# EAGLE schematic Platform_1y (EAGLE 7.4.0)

## Sheet 1 of 5: Propeller
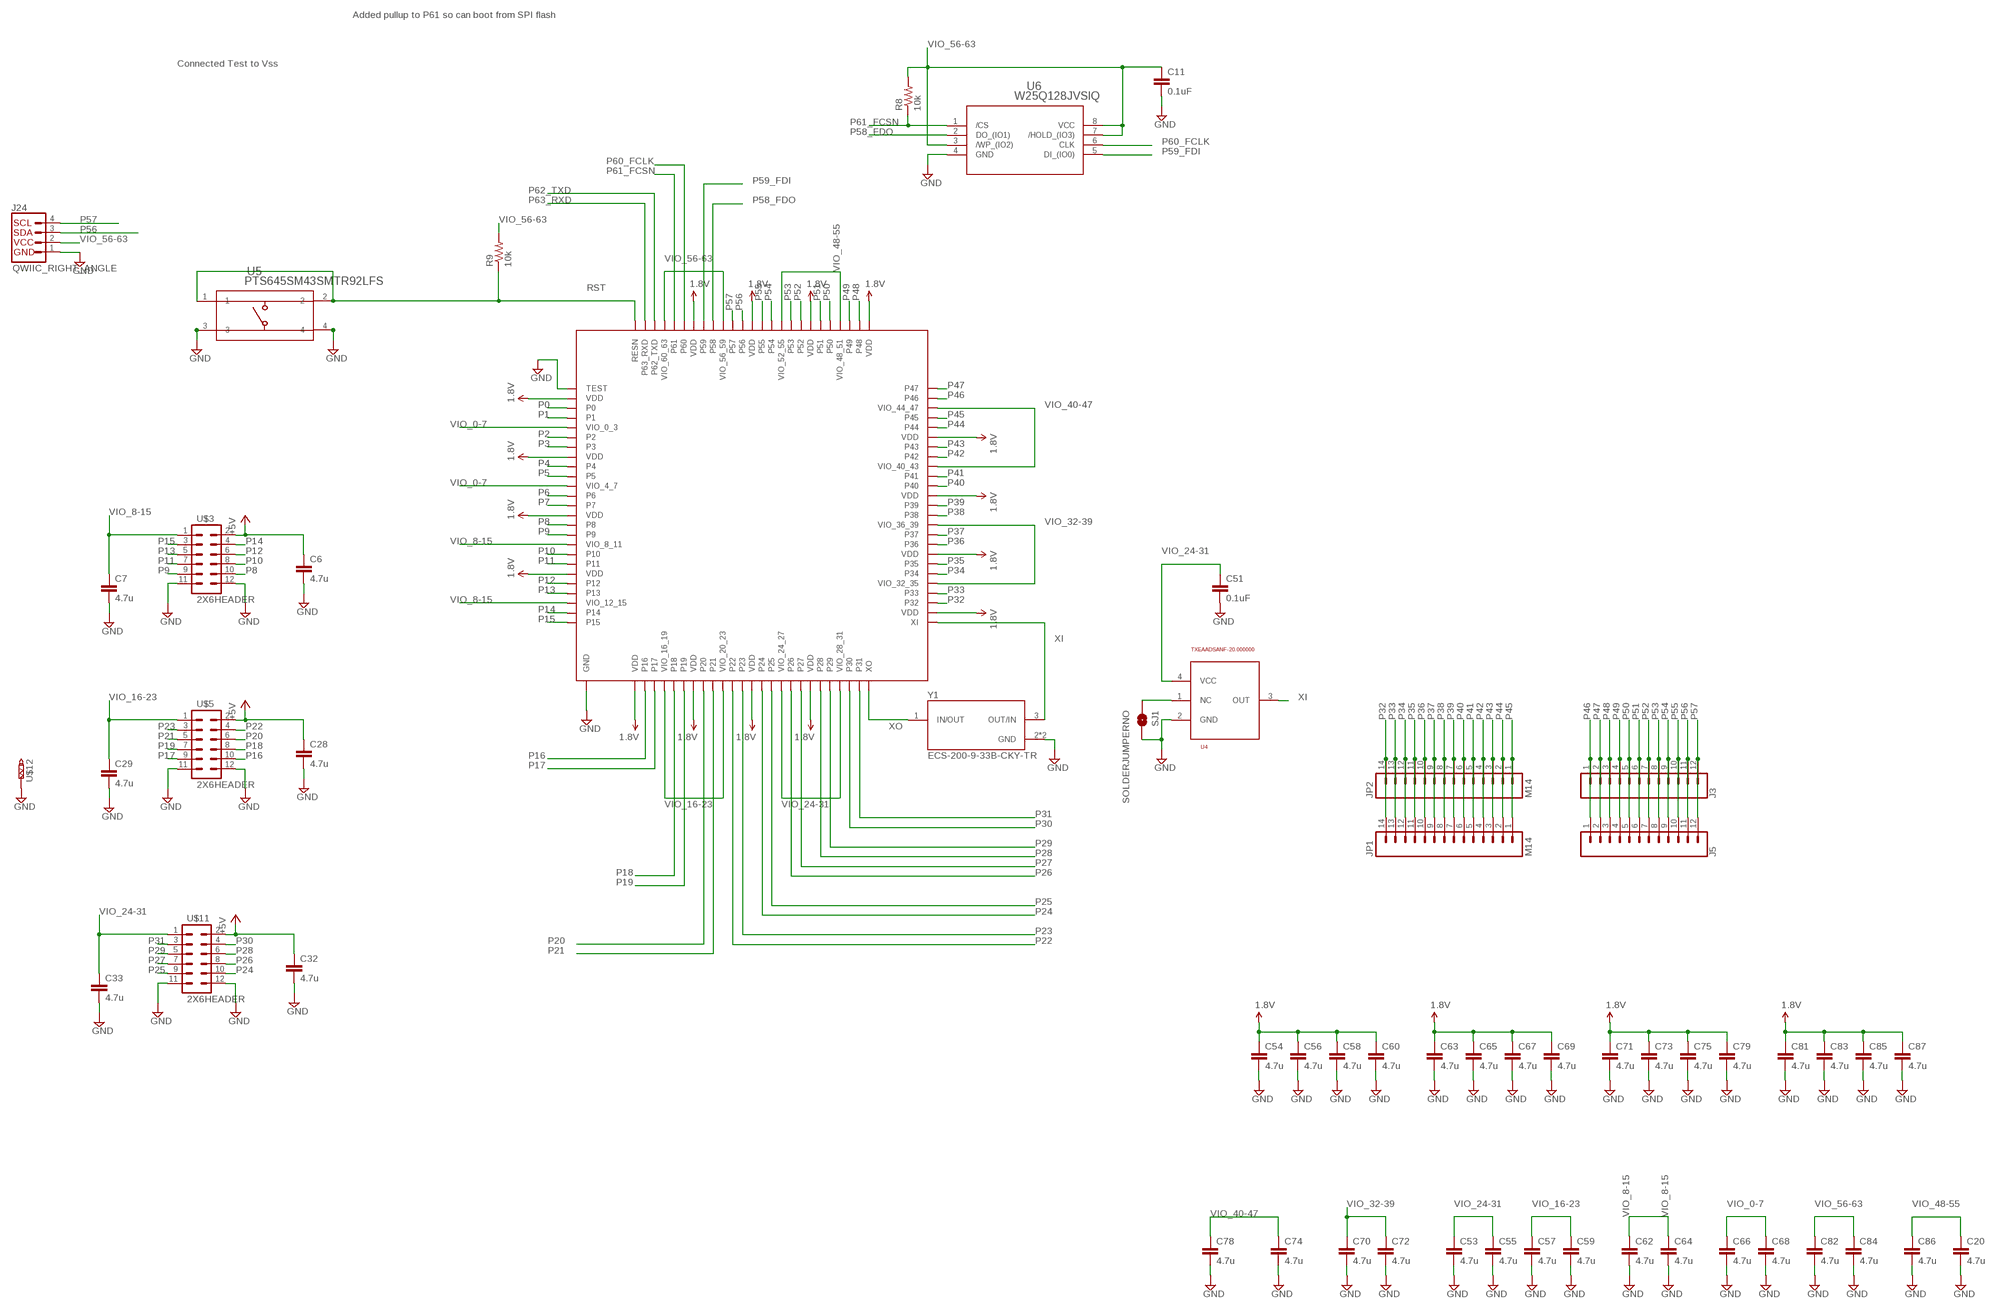
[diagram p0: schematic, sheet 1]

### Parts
C6  4.7u  2.2UF-CERCAP-07888  [0402-CAP]
C7  4.7u  2.2UF-CERCAP-07888  [0402-CAP]
C11  0.1uF  1.0UF-25V-+80/-20(0805)  [0805]
C20  4.7u  2.2UF-CERCAP-07888  [0402-CAP]
C28  4.7u  2.2UF-CERCAP-07888  [0402-CAP]
C29  4.7u  2.2UF-CERCAP-07888  [0402-CAP]
C32  4.7u  2.2UF-CERCAP-07888  [0402-CAP]
C33  4.7u  2.2UF-CERCAP-07888  [0402-CAP]
C51  0.1uF  22UF-6.3V-20%(0805)  [0805]
C53  4.7u  2.2UF-CERCAP-07888  [0402-CAP]
C54  4.7u  2.2UF-CERCAP-07888  [0402-CAP]
C55  4.7u  2.2UF-CERCAP-07888  [0402-CAP]
C56  4.7u  2.2UF-CERCAP-07888  [0402-CAP]
C57  4.7u  2.2UF-CERCAP-07888  [0402-CAP]
C58  4.7u  2.2UF-CERCAP-07888  [0402-CAP]
C59  4.7u  2.2UF-CERCAP-07888  [0402-CAP]
C60  4.7u  2.2UF-CERCAP-07888  [0402-CAP]
C62  4.7u  2.2UF-CERCAP-07888  [0402-CAP]
C63  4.7u  2.2UF-CERCAP-07888  [0402-CAP]
C64  4.7u  2.2UF-CERCAP-07888  [0402-CAP]
C65  4.7u  2.2UF-CERCAP-07888  [0402-CAP]
C66  4.7u  2.2UF-CERCAP-07888  [0402-CAP]
C67  4.7u  2.2UF-CERCAP-07888  [0402-CAP]
C68  4.7u  2.2UF-CERCAP-07888  [0402-CAP]
C69  4.7u  2.2UF-CERCAP-07888  [0402-CAP]
C70  4.7u  2.2UF-CERCAP-07888  [0402-CAP]
C71  4.7u  2.2UF-CERCAP-07888  [0402-CAP]
C72  4.7u  2.2UF-CERCAP-07888  [0402-CAP]
C73  4.7u  2.2UF-CERCAP-07888  [0402-CAP]
C74  4.7u  2.2UF-CERCAP-07888  [0402-CAP]
C75  4.7u  2.2UF-CERCAP-07888  [0402-CAP]
C78  4.7u  2.2UF-CERCAP-07888  [0402-CAP]
C79  4.7u  2.2UF-CERCAP-07888  [0402-CAP]
C81  4.7u  2.2UF-CERCAP-07888  [0402-CAP]
C82  4.7u  2.2UF-CERCAP-07888  [0402-CAP]
C83  4.7u  2.2UF-CERCAP-07888  [0402-CAP]
C84  4.7u  2.2UF-CERCAP-07888  [0402-CAP]
C85  4.7u  2.2UF-CERCAP-07888  [0402-CAP]
C86  4.7u  2.2UF-CERCAP-07888  [0402-CAP]
C87  4.7u  2.2UF-CERCAP-07888  [0402-CAP]
J3  CONN_12  [1X12]
J5  CONN_12  [1X12]
J24  QWIIC_RIGHT_ANGLE  QWIIC_CONNECTORJS-1MM  [JST04_1MM_RA]
JP1  M14  [1X14]
JP2  M14  [1X14]
R8  10k  0.75OHM1/4W1%(0805)  [0805]
R9  10k  0.75OHM1/4W1%(0805)  [0805]
SJ1  SOLDERJUMPERNO  [SJ_2S-NO]
U2  Propeller 2 - ES  P2X8C4M64P-ES_  [PROPELLER_2]
U4  TXEAADSANF-20.000000  [3.2X2.5_4SMD]
U5  PTS645SM43SMTR92LFS  [SWITCH_43SMTR92LFS]
U6  W25Q128JVSIQ  [SOIC_128JVSIQ_WIN]
U$3  2X6HEADER  [6X2HEADER]
U$5  2X6HEADER  [6X2HEADER]
U$11  2X6HEADER  [6X2HEADER]
U$12  TURRET-1520PTH  [1X01_TURRET]
Y1  ECS-200-9-33B-CKY-TR  [XTAL_ECS-200-9-33B-CKY-TR]

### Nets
1.8V: C54.1 C56.1 C58.1 C60.1 C63.1 C65.1 C67.1 C69.1 C71.1 C73.1 C75.1 C79.1 C81.1 C83.1 C85.1 C87.1 U2.2(VDD) U2.8(VDD) U2.14(VDD) U2.20(VDD) U2.26(VDD) U2.32(VDD) U2.38(VDD) U2.44(VDD) U2.52(VDD) U2.58(VDD) U2.64(VDD) U2.70(VDD) U2.76(VDD) U2.82(VDD) U2.88(VDD) U2.94(VDD) ; also sheet 2,4
+5V: C6.1 C28.1 C32.1 U$3.2 U$5.2 U$11.2 ; also sheet 2,4
GND [gnd]: C6.2 C7.2 C11.2 C20.2 C28.2 C29.2 C32.2 C33.2 C51.2 C53.2 C54.2 C55.2 C56.2 C57.2 C58.2 C59.2 C60.2 C62.2 C63.2 C64.2 C65.2 C66.2 C67.2 C68.2 C69.2 C70.2 C71.2 C72.2 C73.2 C74.2 C75.2 C78.2 C79.2 C81.2 C82.2 C83.2 C84.2 C85.2 C86.2 C87.2 J24.1 SJ1.2 U2.1(TEST) U2.EP(GND) U4.2(GND) U5.3 U5.4 U6.4(GND) U$3.11 U$3.12 U$5.11 U$5.12 U$11.11 U$11.12 U$12.1 Y1.2(GND) Y1.4(GND) ; also sheet 2,3,4
N$1 [power]: SJ1.1 U4.1(NC)
P0: U2.3(P0) ; also sheet 3
P1: U2.4(P1) ; also sheet 3
P2: U2.6(P2) ; also sheet 3
P3: U2.7(P3) ; also sheet 3
P4: U2.9(P4) ; also sheet 3
P5: U2.10(P5) ; also sheet 3
P6: U2.12(P6) ; also sheet 3
P7: U2.13(P7) ; also sheet 3
P8: U2.15(P8) U$3.10
P9: U2.16(P9) U$3.9
P10: U2.18(P10) U$3.8
P11: U2.19(P11) U$3.7
P12: U2.21(P12) U$3.6
P13: U2.22(P13) U$3.5
P14: U2.24(P14) U$3.4
P15: U2.25(P15) U$3.3
P16: U2.27(P16) U$5.10
P17: U2.28(P17) U$5.9
P18: U2.30(P18) U$5.8
P19: U2.31(P19) U$5.7
P20: U2.33(P20) U$5.6
P21: U2.34(P21) U$5.5
P22: U2.36(P22) U$5.4
P23: U2.37(P23) U$5.3
P24: U2.39(P24) U$11.10
P25: U2.40(P25) U$11.9
P26: U2.42(P26) U$11.8
P27: U2.43(P27) U$11.7
P28: U2.45(P28) U$11.6
P29: U2.46(P29) U$11.5
P30: U2.48(P30) U$11.4
P31: U2.49(P31) U$11.3
P32: JP1.14 JP2.14 U2.53(P32) ; also sheet 3
P33: JP1.13 JP2.13 U2.54(P33) ; also sheet 3
P34: JP1.12 JP2.12 U2.56(P34) ; also sheet 3
P35: JP1.11 JP2.11 U2.57(P35) ; also sheet 3
P36: JP1.10 JP2.10 U2.59(P36) ; also sheet 3
P37: JP1.9 JP2.9 U2.60(P37) ; also sheet 3
P38: JP1.8 JP2.8 U2.62(P38) ; also sheet 3
P39: JP1.7 JP2.7 U2.63(P39) ; also sheet 3
P40: JP1.6 JP2.6 U2.65(P40) ; also sheet 3
P41: JP1.5 JP2.5 U2.66(P41) ; also sheet 3
P42: JP1.4 JP2.4 U2.68(P42) ; also sheet 3
P43: JP1.3 JP2.3 U2.69(P43) ; also sheet 3
P44: JP1.2 JP2.2 U2.71(P44) ; also sheet 3
P45: JP1.1 JP2.1 U2.72(P45) ; also sheet 3
P46: J3.1 J5.1 U2.74(P46) ; also sheet 3
P47: J3.2 J5.2 U2.75(P47) ; also sheet 3
P48: J3.3 J5.3 U2.77(P48) ; also sheet 3
P49: J3.4 J5.4 U2.78(P49) ; also sheet 3
P50: J3.5 J5.5 U2.80(P50) ; also sheet 3
P51: J3.6 J5.6 U2.81(P51) ; also sheet 3
P52: J3.7 J5.7 U2.83(P52)
P53: J3.8 J5.8 U2.84(P53)
P54: J3.9 J5.9 U2.86(P54)
P55: J3.10 J5.10 U2.87(P55)
P56: J3.11 J5.11 J24.3 U2.89(P56)
P57: J3.12 J5.12 J24.4 U2.90(P57)
P58_FDO: U2.92(P58) U6.2(DO_(IO1))
P59_FDI: U2.93(P59) U6.5(DI_(IO0))
P60_FCLK: U2.95(P60) U6.6(CLK)
P61_FCSN: R8.1 U2.96(P61) U6.1(/CS)
P62_TXD: U2.98(P62_TXD) ; also sheet 2
P63_RXD: U2.99(P63_RXD) ; also sheet 2
RST: R9.1 U2.100(RESN) U5.1 U5.2 ; also sheet 2
VIO_0-7: C66.1 C68.1 U2.5(VIO_0_3) U2.11(VIO_4_7) ; also sheet 3,4
VIO_8-15: C7.1 C62.1 C64.1 U2.17(VIO_8_11) U2.23(VIO_12_15) U$3.1 ; also sheet 4
VIO_16-23: C29.1 C57.1 C59.1 U2.29(VIO_16_19) U2.35(VIO_20_23) U$5.1 ; also sheet 4
VIO_24-31: C33.1 C51.1 C53.1 C55.1 U2.41(VIO_24_27) U2.47(VIO_28_31) U4.4(VCC) U$11.1 ; also sheet 4
VIO_32-39: C70.1 C72.1 U2.55(VIO_32_35) U2.61(VIO_36_39) ; also sheet 3,4
VIO_40-47: C74.1 C78.1 U2.67(VIO_40_43) U2.73(VIO_44_47) ; also sheet 3,4
VIO_48-55: C20.1 C86.1 U2.79(VIO_48_51) U2.85(VIO_52_55) ; also sheet 4
VIO_56-63: C11.1 C82.1 C84.1 J24.2 R8.2 R9.2 U2.91(VIO_56_59) U2.97(VIO_60_63) U6.3(/WP_(IO2)) U6.7(/HOLD_(IO3)) U6.8(VCC) ; also sheet 2,4
XI: U2.51(XI) U4.3(OUT) Y1.3(OUT/IN)
XO: U2.50(XO) Y1.1(IN/OUT)

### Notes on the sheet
- Added pullup to P61 so can boot from SPI flash
- Connected Test to Vss

## Sheet 2 of 5: FT231X
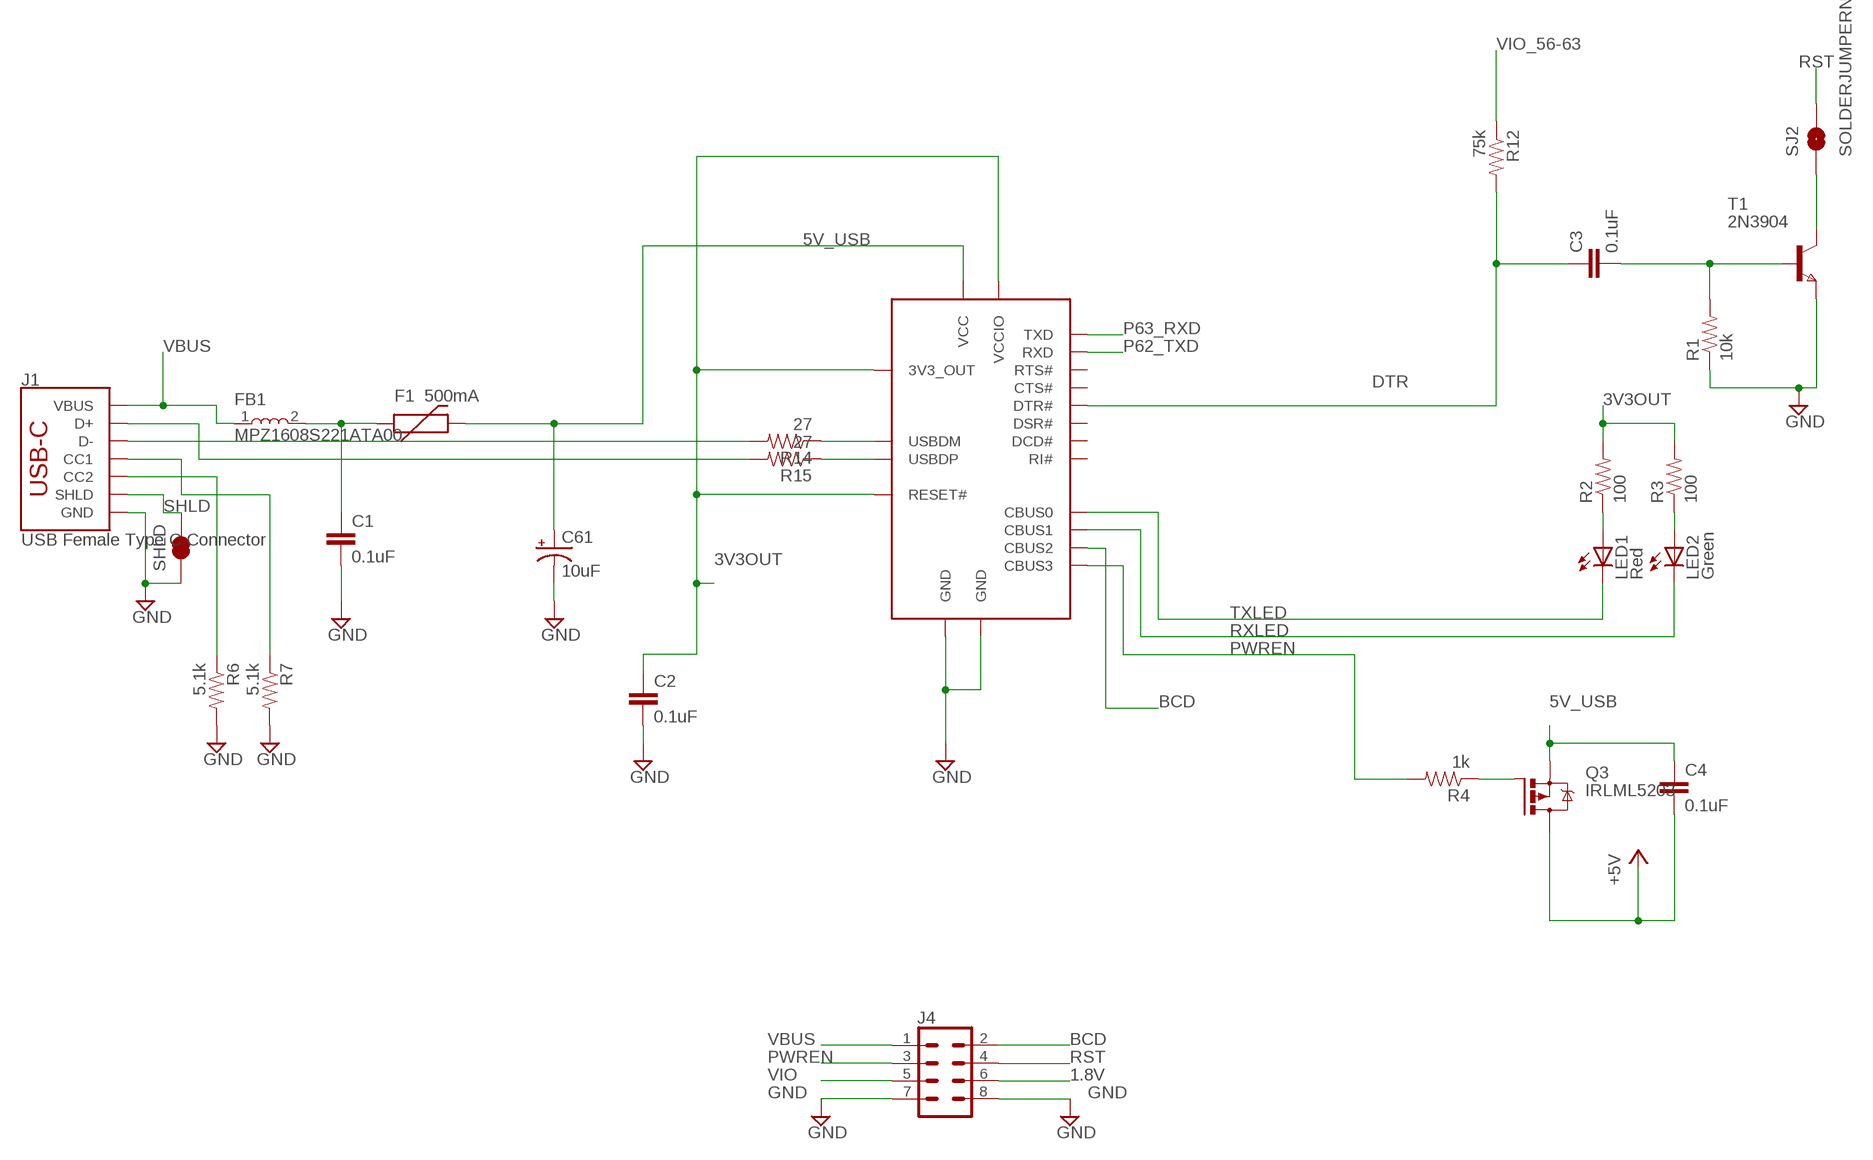
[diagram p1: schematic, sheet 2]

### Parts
C1  0.1uF  1.0UF-25V-+80/-20(0805)  [0805]
C2  0.1uF  1.0UF-25V-+80/-20(0805)  [0805]
C3  0.1uF  1.0UF-25V-+80/-20(0805)  [0805]
C4  0.1uF  1.0UF-25V-+80/-20(0805)  [0805]
C61  10uF  CAP_POL1206  [EIA3216]
F1  500mA  PTCSMD  [PTC-1206]
FB1  MPZ1608S221ATA00  [INDC1608X80]
J1  USB Female Type C Connector  USB_C_4-LAYER-ISOLATED  [USB-C-16P-4LAYER-ISOLATED]
J4  CONN_04X2  [2X4]
LED1  Red  LEDSML0805  [SML0805]
LED2  Green  LEDSML0805  [SML0805]
Q3  IRLML5203  [MICRO3]
R1  10k  0.75OHM1/4W1%(0805)  [0805]
R2  100  0.75OHM1/4W1%(0805)  [0805]
R3  100  0.75OHM1/4W1%(0805)  [0805]
R4  1k  0.75OHM1/4W1%(0805)  [0805]
R6  5.1k  0.75OHM1/4W1%(0805)  [0805]
R7  5.1k  0.75OHM1/4W1%(0805)  [0805]
R12  75k  0.75OHM1/4W1%(0805)  [0805]
R14  27  0.75OHM1/4W1%(0805)  [0805]
R15  27  0.75OHM1/4W1%(0805)  [0805]
SHLD  JUMPER-SMT_2_NC_TRACE_SILK  [SMT-JUMPER_2_NC_TRACE_SILK]
SJ2  SOLDERJUMPERNC  [SJ_2S]
T1  2N3904  NPNSOT23  [SOT-23]
U1  FT231XS-R  604-00065_:_IC-FTDI,_FT231X  [SSOP20]

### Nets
1.8V: J4.6 ; also sheet 1,4
3V3OUT [power]: C2.1 R2.2 R3.2 U1.3(VCCIO) U1.13(3V3_OUT) U1.14(RESET#)
5V_USB [power]: C4.1 C61.A(+) F1.2 Q3.2(S) U1.15(VCC)
+5V: C4.2 Q3.3(D) ; also sheet 1,4
BCD: J4.2 U1.10(CBUS2)
DTR: C3.1 R12.2 U1.1(DTR#)
GND [gnd]: C1.2 C2.2 C61.C(-) J1.GND J1.GND2(GND) J4.7 J4.8 R1.1 R6.2 R7.2 SHLD.1 T1.2(E) U1.6(GND) U1.16(GND) ; also sheet 1,3,4
N$2: LED1.A R2.1
N$4: LED2.A R3.1
N$5: SJ2.1 T1.1(C)
N$6: J1.A5(CC1) R7.1
N$7: J1.B5(CC2) R6.1
N$9: C1.1 F1.1 FB1.2
N$11: R14.1 U1.12(USBDM)
N$12: R15.1 U1.11(USBDP)
N$15: J1.A7(D-) J1.B7(D-) R14.2
N$16: J1.A6(D+) J1.B6(D+) R15.2
N$24: Q3.1(G) R4.1
N$25: C3.2 R1.2 T1.3(B)
P62_TXD: U1.4(RXD) ; also sheet 1
P63_RXD: U1.20(TXD) ; also sheet 1
PWREN: J4.3 R4.2 U1.19(CBUS3)
RST: J4.4 SJ2.2 ; also sheet 1
RXLED: LED2.C U1.17(CBUS1)
SHLD [power]: J1.SHLD1(SHLD) J1.SHLD2(SHLD) J1.SHLD3(SHLD) J1.SHLD4(SHLD) J1.SHLD5(SHLD) J1.SHLD6(SHLD) J1.SHLD7(SHLD) J1.SHLD8(SHLD) SHLD.2
TXLED: LED1.C U1.18(CBUS0)
VBUS: FB1.1 J1.VBUS1(VBUS) J1.VBUS2(VBUS) J4.1
VIO: J4.5 ; also sheet 4
VIO_56-63: R12.1 ; also sheet 1,4
Unconnected: U1.2(RTS#) U1.5(RI#) U1.7(DSR#) U1.8(DCD#) U1.9(CTS#)

## Sheet 3 of 5: Wings
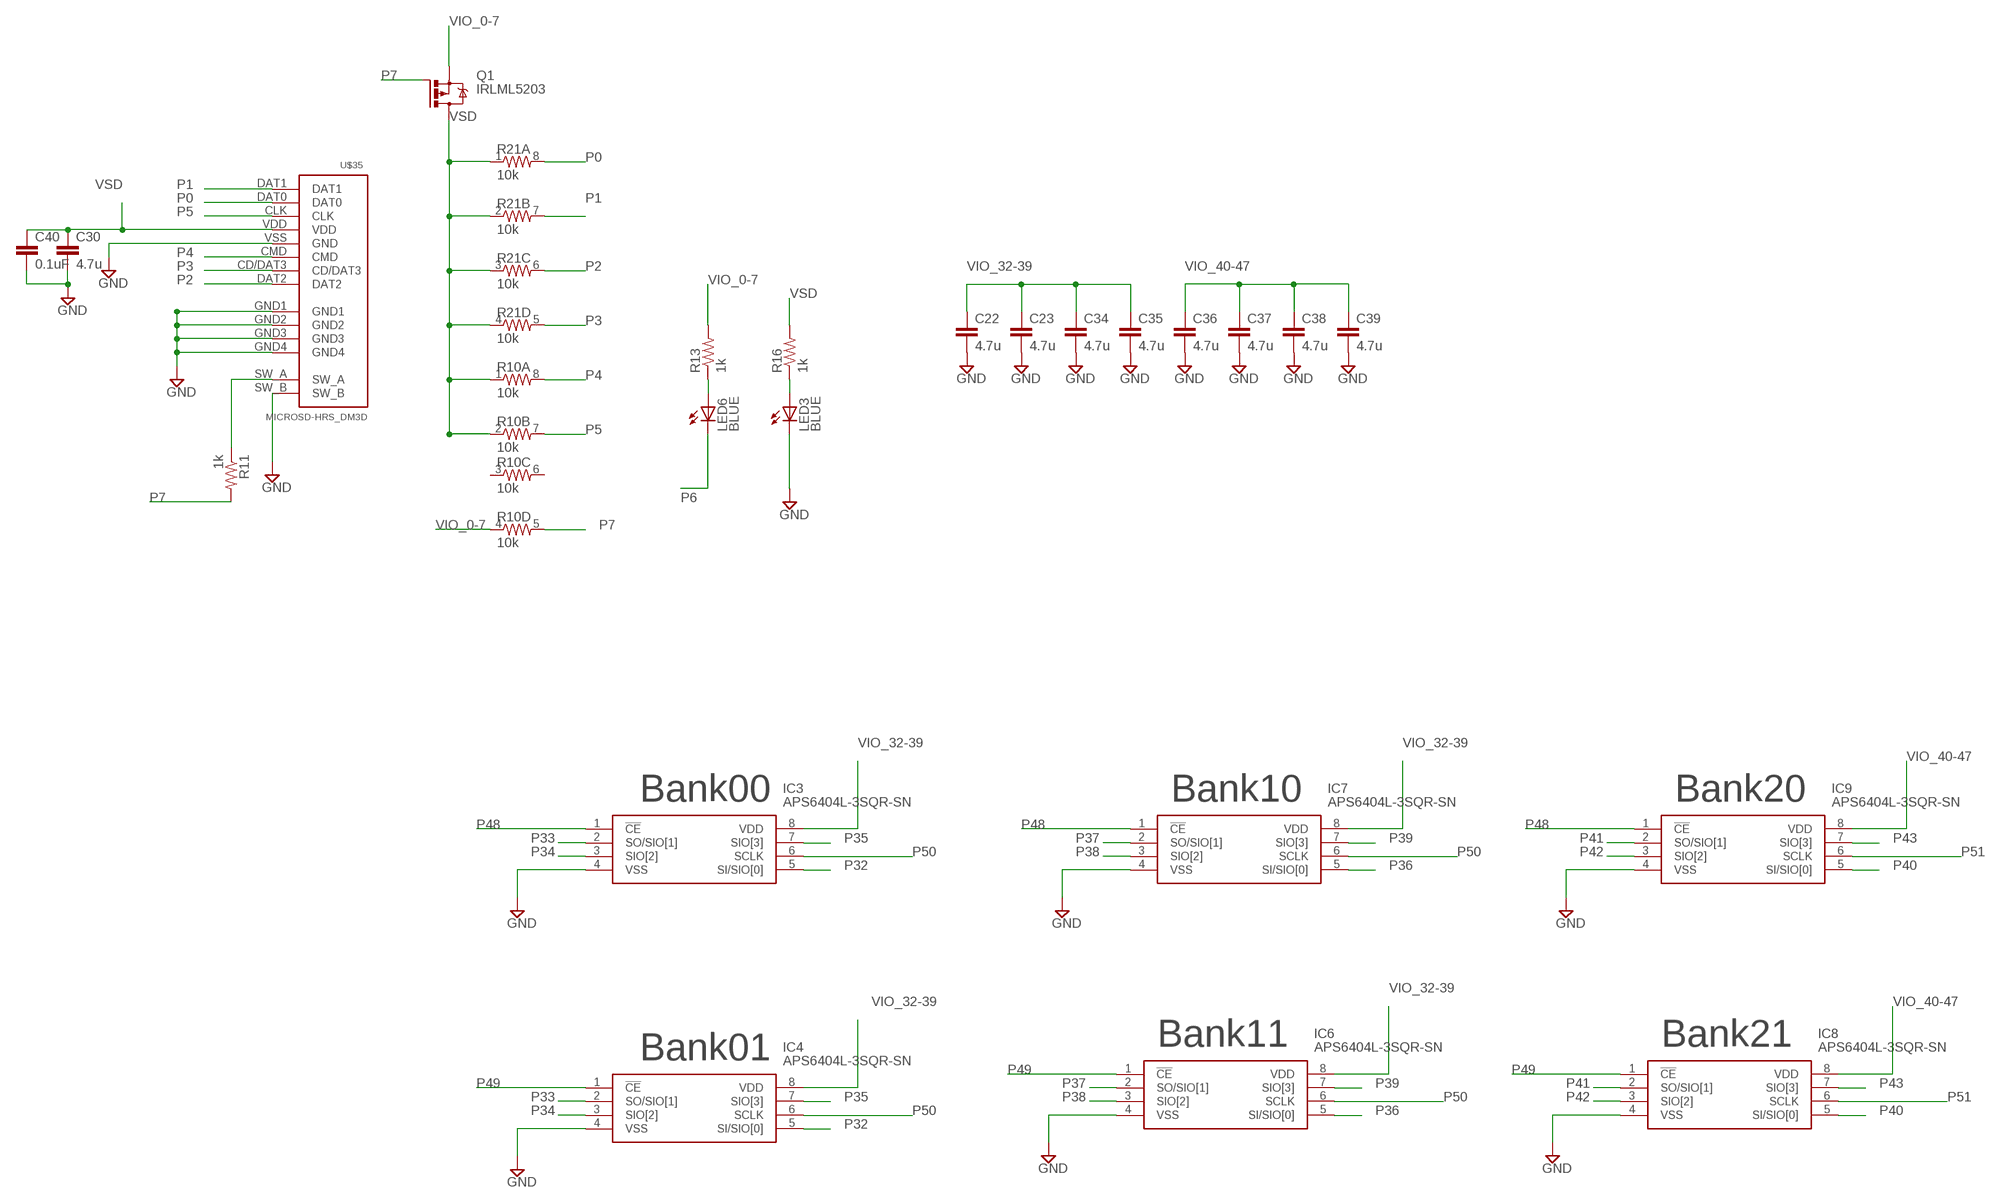
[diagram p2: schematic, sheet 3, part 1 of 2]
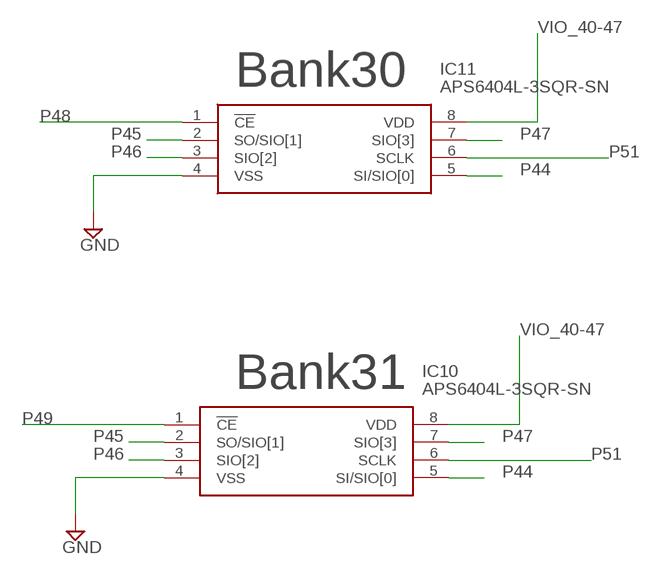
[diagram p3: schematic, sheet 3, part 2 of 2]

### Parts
C22  4.7u  2.2UF-CERCAP-07888  [0402-CAP]
C23  4.7u  2.2UF-CERCAP-07888  [0402-CAP]
C30  4.7u  2.2UF-CERCAP-07888  [0402-CAP]
C34  4.7u  2.2UF-CERCAP-07888  [0402-CAP]
C35  4.7u  2.2UF-CERCAP-07888  [0402-CAP]
C36  4.7u  2.2UF-CERCAP-07888  [0402-CAP]
C37  4.7u  2.2UF-CERCAP-07888  [0402-CAP]
C38  4.7u  2.2UF-CERCAP-07888  [0402-CAP]
C39  4.7u  2.2UF-CERCAP-07888  [0402-CAP]
C40  0.1uF  1.0UF-25V-+80/-20(0805)  [0805]
IC3  APS6404L-3SQR-SN  [SOIC127P600X175-8N]
IC4  APS6404L-3SQR-SN  [SOIC127P600X175-8N]
IC6  APS6404L-3SQR-SN  [SOIC127P600X175-8N]
IC7  APS6404L-3SQR-SN  [SOIC127P600X175-8N]
IC8  APS6404L-3SQR-SN  [SOIC127P600X175-8N]
IC9  APS6404L-3SQR-SN  [SOIC127P600X175-8N]
IC10  APS6404L-3SQR-SN  [SOIC127P600X175-8N]
IC11  APS6404L-3SQR-SN  [SOIC127P600X175-8N]
LED3  BLUE  LEDSML0805  [SML0805]
LED6  BLUE  LEDSML0805  [SML0805]
Q1  IRLML5203  [MICRO3]
R10  10k  RESISTOR-ARRAY0603-ARV  [0603-ARV]
R11  1k  0.75OHM1/4W1%(0805)  [0805]
R13  1k  0.75OHM1/4W1%(0805)  [0805]
R16  1k  0.75OHM1/4W1%(0805)  [0805]
R21  10k  RESISTOR-ARRAY0603-ARV  [0603-ARV]
U$35  MICROSD-HRS_DM3D  [DM3D]

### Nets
GND [gnd]: C22.2 C23.2 C30.2 C34.2 C35.2 C36.2 C37.2 C38.2 C39.2 C40.2 IC3.4(VSS) IC4.4(VSS) IC6.4(VSS) IC7.4(VSS) IC8.4(VSS) IC9.4(VSS) IC10.4(VSS) IC11.4(VSS) LED3.C U$35.GND1 U$35.GND2 U$35.GND3 U$35.GND4 U$35.SW_B U$35.VSS(GND) ; also sheet 1,2,4
N$10: R11.1 U$35.SW_A
N$14: LED3.A R16.1
N$28: LED6.A R13.1
P0: R21.8 U$35.DAT0 ; also sheet 1
P1: R21.7 U$35.DAT1 ; also sheet 1
P2: R21.6 U$35.DAT2 ; also sheet 1
P3: R21.5 U$35.CD/DAT3 ; also sheet 1
P4: R10.8 U$35.CMD ; also sheet 1
P5: R10.7 U$35.CLK ; also sheet 1
P6: LED6.C ; also sheet 1
P7: Q1.1(G) R10.5 R11.2 ; also sheet 1
P32: IC3.5(SI/SIO[0]) IC4.5(SI/SIO[0]) ; also sheet 1
P33: IC3.2(SO/SIO[1]) IC4.2(SO/SIO[1]) ; also sheet 1
P34: IC3.3(SIO[2]) IC4.3(SIO[2]) ; also sheet 1
P35: IC3.7(SIO[3]) IC4.7(SIO[3]) ; also sheet 1
P36: IC6.5(SI/SIO[0]) IC7.5(SI/SIO[0]) ; also sheet 1
P37: IC6.2(SO/SIO[1]) IC7.2(SO/SIO[1]) ; also sheet 1
P38: IC6.3(SIO[2]) IC7.3(SIO[2]) ; also sheet 1
P39: IC6.7(SIO[3]) IC7.7(SIO[3]) ; also sheet 1
P40: IC8.5(SI/SIO[0]) IC9.5(SI/SIO[0]) ; also sheet 1
P41: IC8.2(SO/SIO[1]) IC9.2(SO/SIO[1]) ; also sheet 1
P42: IC8.3(SIO[2]) IC9.3(SIO[2]) ; also sheet 1
P43: IC8.7(SIO[3]) IC9.7(SIO[3]) ; also sheet 1
P44: IC10.5(SI/SIO[0]) IC11.5(SI/SIO[0]) ; also sheet 1
P45: IC10.2(SO/SIO[1]) IC11.2(SO/SIO[1]) ; also sheet 1
P46: IC10.3(SIO[2]) IC11.3(SIO[2]) ; also sheet 1
P47: IC10.7(SIO[3]) IC11.7(SIO[3]) ; also sheet 1
P48: IC3.1(!CE) IC7.1(!CE) IC9.1(!CE) IC11.1(!CE) ; also sheet 1
P49: IC4.1(!CE) IC6.1(!CE) IC8.1(!CE) IC10.1(!CE) ; also sheet 1
P50: IC3.6(SCLK) IC4.6(SCLK) IC6.6(SCLK) IC7.6(SCLK) ; also sheet 1
P51: IC8.6(SCLK) IC9.6(SCLK) IC10.6(SCLK) IC11.6(SCLK) ; also sheet 1
VIO_0-7: Q1.2(S) R10.4 R13.2 ; also sheet 1,4
VIO_32-39: C22.1 C23.1 C34.1 C35.1 IC3.8(VDD) IC4.8(VDD) IC6.8(VDD) IC7.8(VDD) ; also sheet 1,4
VIO_40-47: C36.1 C37.1 C38.1 C39.1 IC8.8(VDD) IC9.8(VDD) IC10.8(VDD) IC11.8(VDD) ; also sheet 1,4
VSD: C30.1 C40.1 Q1.3(D) R10.1 R10.2 R16.2 R21.1 R21.2 R21.3 R21.4 U$35.VDD
Unconnected: R10.3 R10.6

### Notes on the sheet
- Bank00 | Bank10 | Bank20 | Bank30
- Bank31
- Bank11 | Bank21
- Bank01

## Sheet 4 of 5: Power
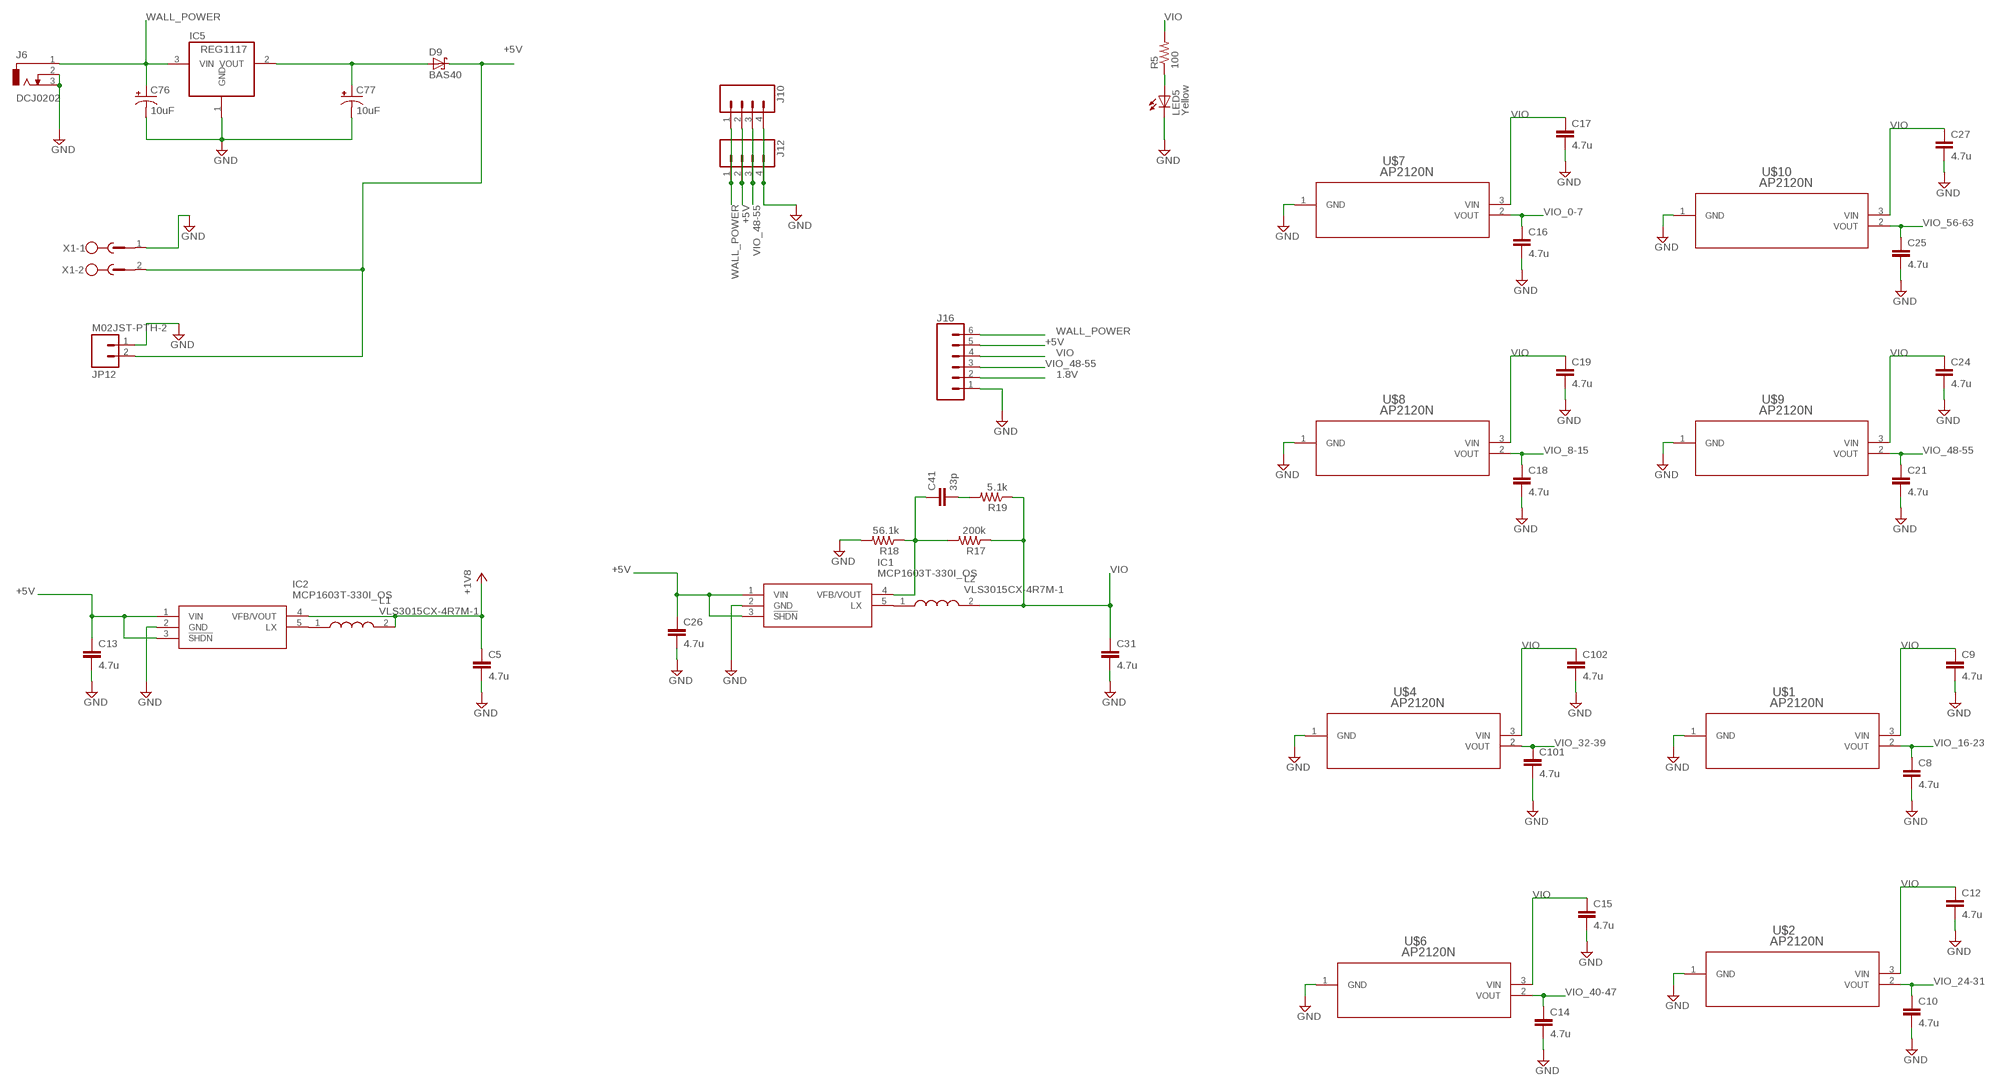
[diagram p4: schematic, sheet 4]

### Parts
C5  4.7u  C-EUC0805  [C0805]
C8  4.7u  2.2UF-CERCAP-07888  [0402-CAP]
C9  4.7u  2.2UF-CERCAP-07888  [0402-CAP]
C10  4.7u  2.2UF-CERCAP-07888  [0402-CAP]
C12  4.7u  2.2UF-CERCAP-07888  [0402-CAP]
C13  4.7u  C-EUC0805  [C0805]
C14  4.7u  2.2UF-CERCAP-07888  [0402-CAP]
C15  4.7u  2.2UF-CERCAP-07888  [0402-CAP]
C16  4.7u  2.2UF-CERCAP-07888  [0402-CAP]
C17  4.7u  2.2UF-CERCAP-07888  [0402-CAP]
C18  4.7u  2.2UF-CERCAP-07888  [0402-CAP]
C19  4.7u  2.2UF-CERCAP-07888  [0402-CAP]
C21  4.7u  2.2UF-CERCAP-07888  [0402-CAP]
C24  4.7u  2.2UF-CERCAP-07888  [0402-CAP]
C25  4.7u  2.2UF-CERCAP-07888  [0402-CAP]
C26  4.7u  C-EUC0805  [C0805]
C27  4.7u  2.2UF-CERCAP-07888  [0402-CAP]
C31  4.7u  C-EUC0805  [C0805]
C41  33p  1.0UF-25V-+80/-20(0805)  [0805]
C76  10uF  10UF-16V-10%(TANT)  [EIA3216]
C77  10uF  10UF-16V-10%(TANT)  [EIA3216]
C101  4.7u  2.2UF-CERCAP-07888  [0402-CAP]
C102  4.7u  2.2UF-CERCAP-07888  [0402-CAP]
D9  BAS40  [SOT23]
IC1  MCP1603T-330I_OS  [SOT95P280X110-5N]
IC2  MCP1603T-330I_OS  [SOT95P280X110-5N]
IC5  REG1117  [SOT223]
J6  DCJ0202  [DCJ0202]
J10  CONN_04PTH  [1X04]
J12  CONN_04PTH  [1X04]
J16  CONN_06LONGPADS  [1X06_LONGPADS]
JP12  M02JST-PTH-2  [JST-2-PTH]
L1  VLS3015CX-4R7M-1  [VLS3015]
L2  VLS3015CX-4R7M-1  [VLS3015]
LED5  Yellow  LEDSML0805  [SML0805]
R5  100  0.75OHM1/4W1%(0805)  [0805]
R17  200k  0.75OHM1/4W1%(0805)  [0805]
R18  56.1k  0.75OHM1/4W1%(0805)  [0805]
R19  5.1k  0.75OHM1/4W1%(0805)  [0805]
U$1  AP2120N  [SOT-23_DIO]
U$2  AP2120N  [SOT-23_DIO]
U$4  AP2120N  [SOT-23_DIO]
U$6  AP2120N  [SOT-23_DIO]
U$7  AP2120N  [SOT-23_DIO]
U$8  AP2120N  [SOT-23_DIO]
U$9  AP2120N  [SOT-23_DIO]
U$10  AP2120N  [SOT-23_DIO]
X1  MSTBV2  [MSTBV2]

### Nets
1.8V: C5.1 IC2.4(VFB/VOUT) J16.2 L1.2 ; supply symbol labelled +1V8 ; also sheet 1,2
+5V: C13.1 C26.1 D9.3(C) IC1.1(VIN) IC1.3(!SHDN) IC2.1(VIN) IC2.3(!SHDN) J10.2 J12.2 J16.5 JP12.2 X1.2 ; also sheet 1,2
GND [gnd]: C5.2 C8.2 C9.2 C10.2 C12.2 C13.2 C14.2 C15.2 C16.2 C17.2 C18.2 C19.2 C21.2 C24.2 C25.2 C26.2 C27.2 C31.2 C76.C(-) C77.C(-) C101.2 C102.2 IC1.2(GND) IC2.2(GND) IC5.1(GND) J6.2 J6.3 J10.4 J12.4 J16.1 JP12.1 LED5.C R18.2 U$1.1(GND) U$2.1(GND) U$4.1(GND) U$6.1(GND) U$7.1(GND) U$8.1(GND) U$9.1(GND) U$10.1(GND) X1.1 ; also sheet 1,2,3
N$8: C41.2 R19.2
N$13: C77.A(+) D9.1(A) IC5.2(VOUT)
N$17: IC2.5(LX) L1.1
N$18: C41.1 IC1.4(VFB/VOUT) R17.2 R18.1
N$19: IC1.5(LX) L2.1
N$45: LED5.A R5.1
VIO: C9.1 C12.1 C15.1 C17.1 C19.1 C24.1 C27.1 C31.1 C102.1 J16.4 L2.2 R5.2 R17.1 R19.1 U$1.3(VIN) U$2.3(VIN) U$4.3(VIN) U$6.3(VIN) U$7.3(VIN) U$8.3(VIN) U$9.3(VIN) U$10.3(VIN) ; also sheet 2
VIO_0-7: C16.1 U$7.2(VOUT) ; also sheet 1,3
VIO_8-15: C18.1 U$8.2(VOUT) ; also sheet 1
VIO_16-23: C8.1 U$1.2(VOUT) ; also sheet 1
VIO_24-31: C10.1 U$2.2(VOUT) ; also sheet 1
VIO_32-39: C101.1 U$4.2(VOUT) ; also sheet 1,3
VIO_40-47: C14.1 U$6.2(VOUT) ; also sheet 1,3
VIO_48-55: C21.1 J10.3 J12.3 J16.3 U$9.2(VOUT) ; also sheet 1
VIO_56-63: C25.1 U$10.2(VOUT) ; also sheet 1,2
WALL_POWER: C76.A(+) IC5.3(VIN) J6.1 J10.1 J12.1 J16.6

## Sheet 5 of 5: Extra

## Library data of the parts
C1-C4 C11 C40 C41 = SparkFun-Capacitors:1.0UF-25V-+80/-20(0805); PROD_ID: CAP-11625; VALUE: 1.0uF
C5 C13 C26 C31 = rcl:C-EU: CAPACITOR, European symbol
C6-C10 C12 C14-C25 C27-C30 C32-C39 C53-C60 C62-C75 C78 C79 C81-C87 C101 C102 = SparkFun-Capacitors:2.2UF-CER: 2.2uF Ceramic SMT; PROD_ID: CAP-07888; VALUE: 2.2uF
C51 = SparkFun-Capacitors:22UF-6.3V-20%(0805): Ceramic; PROD_ID: CAP-08402; VALUE: 22uF
C61 = SparkFun:CAP_POL: Capacitor Polarized
C76 C77 = SparkFun-Capacitors:10UF-16V-10%(TANT): CAP-00811; PROD_ID: CAP-00811
D9 = diode:BAS40: Silicon Schottky Diodes
F1 = SparkFun:PTC: Resettable Fuse PTC
FB1 = ray2:MPZ1608S221ATA00: Ind Chip Bead Multi-Layer 220Ohm 25% 100MHz Ferrite 2.2A 0603 Punched Paper T/R; DESCRIPTION: Ind Chip Bead Multi-Layer 220Ohm 25% 100MHz Ferrite 2.2A 0603 Punched Paper T/R; DIGI-KEY_PART_NUMBER: 445-1565-1-ND; DIGI-KEY_PURCHASE_URL: https://www.digikey.com/product-detail/en/tdk-corporation/MPZ1608S221ATA00/445-1565-1-ND/571895?utm_source=snapeda&utm_medium=aggregator&utm_campaign=symbol; MF: TDK; MP: MPZ1608S221ATA00; PACKAGE: 0603 TDK
IC1 IC2 = SamacSys_Parts:MCP1603T-330I_OS: Sw. Reg. PWM/PFM 2MHz 500mA 3.3V TSOT5 Source: Datasheet; DESCRIPTION: Sw. Reg. PWM/PFM 2MHz 500mA 3.3V TSOT5; HEIGHT: 1.1mm; MANUFACTURER_NAME: Microchip; MANUFACTURER_PART_NUMBER: MCP1603T-330I/OS; MOUSER_PART_NUMBER: 579-MCP1603T-330I/OS; MOUSER_PRICE-STOCK: https://www.mouser.co.uk/ProductDetail/Microchip-Technology-Atmel/MCP1603T-330I-OS?qs=usxtMOJb1RzTHtIF7bKmHg%3D%3D
IC3 IC4 IC6-IC11 = SamacSys_Parts:APS6404L-3SQR-SN: DRAM IoT RAM 64Mb QSPI (x1,x4) SDR 133/84MHz, RBX, 3V, Ind. Temp., SOP8 Source: Datasheet; DESCRIPTION: DRAM IoT RAM 64Mb QSPI (x1,x4) SDR 133/84MHz, RBX, 3V, Ind. Temp., SOP8; HEIGHT: 1.75mm; MANUFACTURER_NAME: AP Memory; MANUFACTURER_PART_NUMBER: APS6404L-3SQR-SN; MOUSER_PART_NUMBER: 878-APS6404L-3SQR-SN; MOUSER_PRICE-STOCK: https://www.mouser.co.uk/ProductDetail/AP-Memory/APS6404L-3SQR-SN?qs=IS%252B4QmGtzzqsn3S5xo%2FEEg%3D%3D
IC5 = burr-brown:REG1117: 800mA and 1A Low Dropout (LDO) Positive Regulator 1.8V, 2.5V, 2.85V, 3.3V, 5V, and Adj; MPN: REG1117; OC_FARNELL: 1097566; OC_NEWARK: 14P6981
J1 = SparkFun-Connectors:USB_C: USB Type C 16Pin Connector Super Speed pins not available on the 16-pin purely SMD connector so this part is best for USB 2.0 implementations. D1 and D2 are tied together enabling D+/- no matter which way the cable is plugged into the connector. The two channel configuration pins (CC1/2) are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; PROD_ID: CONN-14122
J3 J5 = SparkFun-Connectors:CONN_12: Multi connection point. Often used as Generic Header-pin footprint for 0.1 inch spaced/style header connections On any of the 0.1 inch spaced packages, you can populate with these: Break Away Headers - Straight (PRT-00116) Break Away Male Headers - Right Angle (PRT-00553) Female Headers (PRT-00115)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
J4 = SparkFun-Connectors:CONN_04X2: Multi connection point. Often used as Generic Header-pin footprint for 0.1 inch spaced/style header connections On any of the 0.1 inch spaced packages, you can populate with these: Break Away Headers - Straight (PRT-00116) Break Away Male Headers - Right Angle (PRT-00553) Female Headers (PRT-00115)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
J6 = con-jack:DCJ0202: DC POWER JACK Source: DCJ0202.pdf; OC_FARNELL: unknown; OC_NEWARK: unknown
J10 J12 = SparkFun-Connectors:CONN_04: Multi connection point. Often used as Generic Header-pin footprint for 0.1 inch spaced/style header connections On any of the 0.1 inch spaced packages, you can populate with these: Break Away Headers - Straight (PRT-00116) Break Away Male Headers - Right Angle (PRT-00553) Female Headers (PRT-00115)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; PROD_ID: CONN-09696
J16 = SparkFun-Connectors:CONN_06: Multi connection point. Often used as Generic Header-pin footprint for 0.1 inch spaced/style header connections On any of the 0.1 inch spaced packages, you can populate with these: Break Away Headers - Straight (PRT-00116) Break Away Male Headers - Right Angle (PRT-00553) Female Headers (PRT-00115)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
J24 = SparkFun-Connectors:QWIIC_CONNECTOR: SparkFun I2C Standard Qwiic Connector An SMD 1mm pitch JST connector makes it easy and quick (get it? Qwiic?) to connect I2C devices to each other. The Qwiic system enables fast and solderless connection between popular platforms and various sensors and actuators. We carry 200mm, 100mm, 50mm, and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; PROD_ID: CONN-13694
JP1 JP2 = SparkFun-Connectors:M14: Header 14 Standard 14-pin 0.1" header. Use with straight break away headers (SKU : PRT-00116), right angle break away headers (PRT-00553), swiss pins (PRT-00743), machine pins (PRT-00117), and female headers (PRT-00115).
JP12 = SparkFun-Connectors:M02: Standard 2-pin 0.1" header. Use with
L1 L2 = SamacSys_Parts:VLS3015CX-4R7M-1: SMD / SMT Inductors (Coils), L=4.7?H, L x W x T :; DESCRIPTION: SMD / SMT Inductors (Coils), L=4.7?H, L x W x T :; HEIGHT: mm; MANUFACTURER_NAME: TDK; MANUFACTURER_PART_NUMBER: VLS3015CX-4R7M-1; MOUSER_PART_NUMBER: 810-VLS3015CX-4R7M-1; MOUSER_PRICE-STOCK: https://www.mouser.co.uk/ProductDetail/TDK/VLS3015CX-4R7M-1?qs=gZXFycFWdANzf31QH9GBWA%3D%3D
LED1-LED3 LED5 LED6 = led:LED: LED
Q1 Q3 = transistor-power:IRLML5203: HEXFET P-Channel Power MOSFET
R1-R9 R11-R19 = SparkFun-Resistors:0.75OHM1/4W1%(0805): RES-08474; PROD_ID: RES-08474; VALUE: 0.75
R10 R21 = SparkFun-Passives:RESISTOR-ARRAY: Array Chip Resistor Source: RS Component / Phycomp
SHLD = SparkFun-Jumpers:JUMPER-SMT_2_NC_TRACE: Normally closed trace jumper
SJ1 SJ2 = SparkFun-Passives:SOLDERJUMPER: Solder Jumper
T1 = zetex:NPNSOT23: NPN TRANSISTOR; MPN: DSS20201L-7; OC_FARNELL: 1710688; OC_NEWARK: 25R4555
U1 = ray2:604-00065_:_IC-FTDI,_FT231X; MANUFACTURER: FTDI : FT231XS-R; POPULATED: True
U2 = ray2:P2X8C4M64P-ES_; MANUFACTURER: Parallax : P2X8C4M64P-ES
U4 = ray2:TXEAADSANF-20.000000: 20MHz VCTCXO Clipped Sine Wave Oscillator 2.8 V ~ 3.3 V 4-SMD, No Lead Check availability; AVAILABILITY: In Stock; DESCRIPTION: 20 MHz VCTCXO Clipped Sine Wave Oscillator 2.8V ~ 3.3V - 4-SMD, No Lead; MF: Taitien; MP: TXEAADSANF-20.000000; PACKAGE: SMD-4 Taitien; PRICE: None; PURCHASE-URL: https://pricing.snapeda.com/search/part/TXEAADSANF-20.000000/?ref=eda
U5 = ray2:PTS645SM43SMTR92LFS; COPYRIGHT: Copyright (C) 2024 Ultra Librarian. All rights reserved.; MANUFACTURER_PART_NUMBER: PTS645SM43SMTR92LFS; MFR_NAME: C&K Components
U6 = ray2:W25Q128JVSIQ; COPYRIGHT: Copyright (C) 2024 Ultra Librarian. All rights reserved.; MANUFACTURER_PART_NUMBER: W25Q128JVSIQ; MFR_NAME: Winbond
U$1 U$2 U$4 U$6-U$10 = ray2:AP2120N
U$3 U$5 U$11 = ray2:2X6HEADER
U$12 = SparkFun-Electromechanical:TURRET-1520: Turret FP for Keystone Electronics Part#1520
U$35 = hrs_DM3D-SF:MICROSD-HRS_DM3D
X1 = con-phoenix-500:MSTBV2: PHOENIX; OC_FARNELL: unknown; OC_NEWARK: unknown
Y1 = ray2:ECS-200-9-33B-CKY-TR: The miniature ECS-33B is a compact SMD Crystal. The industry standard 3.2 x 2.5 x 0.8 mm ceramic package is ideal for today’s wireless applications.; DESCRIPTION: CRYSTAL 20MHZ 9PF SMD; DIGI-KEY_PART_NUMBER: XC2464CT-ND; DIGI-KEY_PURCHASE_URL: https://www.digikey.com/product-detail/en/ecs-inc/ECS-200-9-33B-CKY-TR/XC2464CT-ND/8023399?utm_source=snapeda&utm_medium=aggregator&utm_campaign=symbol; MF: ECS Inc.; MP: ECS-200-9-33B-CKY-TR; PACKAGE: SMD-4 ECS Inc.

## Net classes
0 default: width 0.203 mm, drill 0.406 mm, clearance 0.203 mm
1 power: width 0.254 mm
2 gnd: width 0.305 mm, drill 0.406 mm, clearance 0.203 mm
